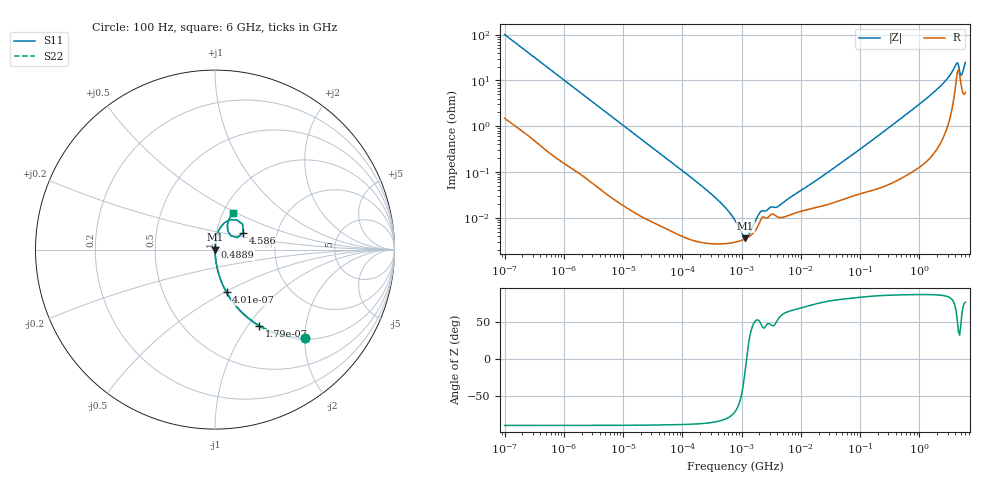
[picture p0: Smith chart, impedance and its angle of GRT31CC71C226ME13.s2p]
!Murata Part Number: GRT31CC71C226ME13
!These Parameters are Measured in Series Mode Connection
!Data Generated on Jun 19, 2026
!  o--ll--o
!Port1  Port2
!  o------o
!Operation Temp=25[degC], DC Bias Voltage=0[V]
!Freq. Start=100[Hz] Stop=6[GHz] 401[Steps]
# Hz S RI R 50
!Freq.(Hz) S11(Real) S11(Imag) S21(Real) S21(Imag) S12(Real) S12(Imag) S22(Real) S22(Imag)
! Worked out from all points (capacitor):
!   401 points, 100 Hz to 6 GHz, reference 50 ohm
!   read as one part in series: C = 15.7 uF near 109 Hz
!   lowest |Z| = 3.59 mohm at 1.159 MHz (marker M1)
!   series resonance near 1.211 MHz, so ESL is about 1.1 nH
!   S11 on the Smith chart (normalised r, x): 100 Hz: 1.03, -2.02; 179 Hz: 1.02, -1.13; 401 Hz: 1.01, -0.51; 488.9 MHz: 1.00, +0.03; 4.586 GHz: 1.35, +0.26; 6 GHz: 1.11, +0.48
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100  0.5038 -0.4926  0.4962 0.4926  0.4962 0.4926  0.5038 -0.4926
179  0.246 -0.4231  0.754 0.4231  0.754 0.4231  0.246 -0.4231
401  0.0641 -0.2377  0.9359 0.2377  0.9359 0.2377  0.0641 -0.2377
820  0.0172 -0.1229  0.9828 0.1229  0.9828 0.1229  0.0172 -0.1229
2008  0.0035 -0.0514  0.9965 0.0514  0.9965 0.0514  0.0035 -0.0514
40335  7.6e-05 -0.00265  0.9999 0.00265  0.9999 0.00265  7.6e-05 -0.00265
276587  2.78e-05 -0.000373  1 0.000373  1 0.000373  2.78e-05 -0.000373
774597  2.94e-05 -8.38e-05  1 8.38e-05  1 8.38e-05  2.94e-05 -8.38e-05
1159002  3.5e-05 -8e-06  1 8e-06  1 8e-06  3.5e-05 -8e-06
1658239  5.04e-05 6.13e-05  0.9999 -6.13e-05  0.9999 -6.13e-05  5.04e-05 6.13e-05
2169299  9.83e-05 0.000103  0.9999 -0.000103  0.9999 -0.000103  9.83e-05 0.000103
4060267  0.000105 0.000141  0.9999 -0.000141  0.9999 -0.000141  0.000105 0.000141
1.555665e7  0.000161 0.000551  0.9998 -0.000551  0.9998 -0.000551  0.000161 0.000551
3.124326e8  0.000631 0.00948  0.9994 -0.00948  0.9994 -0.00948  0.000631 0.00948
4.888888e8  0.000939 0.0147  0.9991 -0.0147  0.9991 -0.0147  0.000939 0.0147
2.048624e9  0.00766 0.0654  0.9923 -0.0654  0.9923 -0.0654  0.00766 0.0654
3.205649e9  0.0275 0.1185  0.9725 -0.1185  0.9725 -0.1185  0.0275 0.1185
4.009986e9  0.0885 0.1667  0.9115 -0.1667  0.9115 -0.1667  0.0885 0.1667
4.193612e9  0.1204 0.1657  0.8796 -0.1657  0.8796 -0.1657  0.1204 0.1657
4.586474e9  0.158 0.0937  0.842 -0.0937  0.842 -0.0937  0.158 0.0937
5.245841e9  0.0712 0.1042  0.9288 -0.1042  0.9288 -0.1042  0.0712 0.1042
6e9  0.0995 0.2065  0.9005 -0.2065  0.9005 -0.2065  0.0995 0.2065
